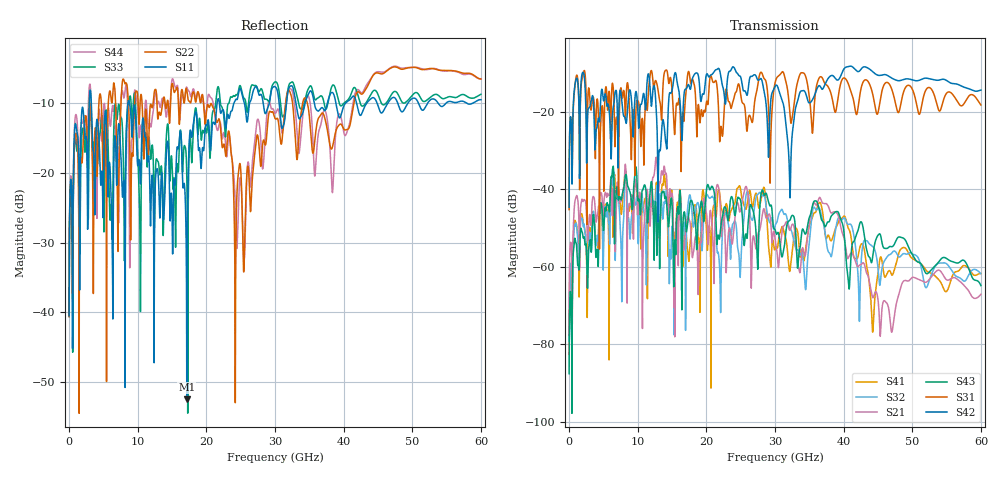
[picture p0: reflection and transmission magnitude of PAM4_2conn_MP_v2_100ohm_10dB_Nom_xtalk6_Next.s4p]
! Info: Touchstone file created by Circ.  Input file=FAB50GbE_2conn_Midplane_Examax_Topo2_v2_100ohm_10dB_Nom.circ
# Hz S RI R 50
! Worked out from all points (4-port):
!   6000 points, 10 MHz to 60 GHz, reference 50 ohm
!   strongest paths, dB at 10 MHz, 15.01 GHz, 30.01 GHz, 45.01 GHz, 60 GHz:
!     S42: -44.6, -14.5, -13.5, -10.6, -14.4
!     S31: -45.2, -14.6, -12.6, -20.2, -18.3
!     S43: -87.5, -43.9, -50.4, -51.8, -64.8
!     S21: -77.6, -41.2, -52.7, -68.4, -67.1
!     S32: -79.1, -49.7, -49.4, -60.3, -61.8
!     S41: -82.6, -40.9, -55.5, -61.6, -61.7
!   lowest |S11| = -52.5 dB at 17.15 GHz (marker M1), VSWR 1.00, Z = 49.8 - j0.0519 ohm
!   |S11| at or under -10 dB: start of sweep to 2.94 GHz; 3.243 GHz to 8.574 GHz (5.331 GHz wide, 90.2 % of centre); 8.802 GHz to 21.57 GHz (12.77 GHz wide, 84.1 % of centre)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
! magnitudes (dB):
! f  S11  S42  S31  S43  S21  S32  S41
! 10 MHz  -40.5  -44.6  -45.2  -87.5  -77.6  -79.1  -82.6
! 1.04 GHz  -13.4  -11.6  -10.9  -53.9  -41.8  -48.8  -48.8
! 6.27 GHz  -29.5  -23.3  -13.1  -36.1  -44.8  -39.0  -40.0
! 17.15 GHz  -52.5  -13.9  -12.7  -50.4  -47.9  -48.6  -53.4
! 25.48 GHz  -9.8  -14.6  -18.0  -54.1  -40.9  -47.2  -44.0
! 44.24 GHz  -9.2  -9.7  -15.5  -57.4  -67.9  -54.8  -76.8
! 60 GHz  -9.5  -14.4  -18.3  -64.8  -67.1  -61.8  -61.7
